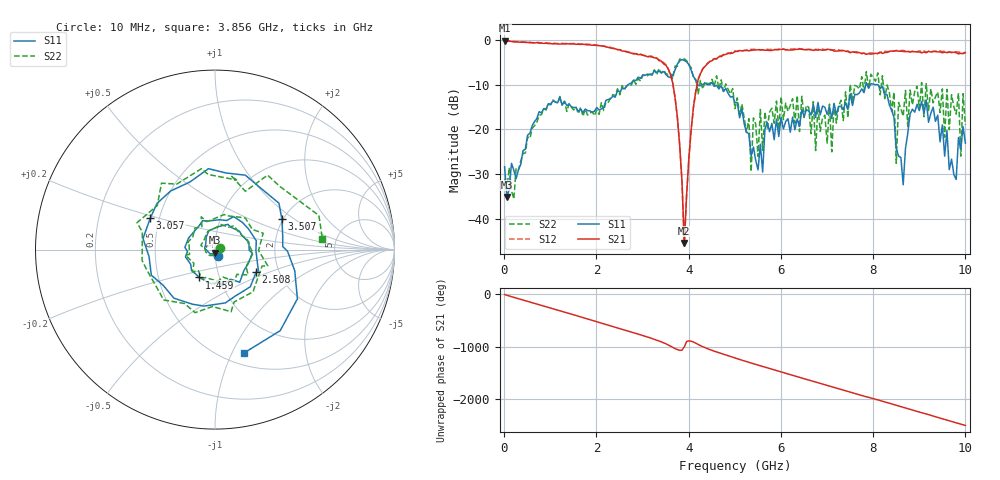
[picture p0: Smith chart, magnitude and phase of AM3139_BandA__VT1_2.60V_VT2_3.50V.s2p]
! Date/Time: Tue, Nov 13, 2018 4:57 PM
! Network Analyzer: Agilent Technologies E8364B Rev: A.07.50.67
! Sweep from 0.010 to 10.000 GHz, 201 Points, Sweep Type: LIN
! Power Supply: 2.601 V, 0.000 A
# Hz S DB R 50
!freq MagS11 AngS11 MagS21 AngS21 MagS12 AngS12 MagS22 AngS22
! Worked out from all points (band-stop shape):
!   201 points, 10 MHz to 10 GHz, reference 50 ohm
!   highest |S21| = -0.23 dB at 10 MHz (marker M1); lowest = -45.3 dB at 3.906 GHz (marker M2)
!   |S21| within 3 dB of the highest: start of sweep to 2.874 GHz; 4.816 GHz to 7.843 GHz (3.027 GHz wide, 47.8 % of centre)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
!   lowest |S11| = -35.1 dB at 59.95 MHz (marker M3), VSWR 1.04, Z = 49.8 - j1.75 ohm
!   |S11| at or under -10 dB: start of sweep to 2.696 GHz; 4.531 GHz to 7.843 GHz (3.312 GHz wide, 53.5 % of centre); 8.036 GHz to end of sweep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
!   |S22| runs from -35.5 to -4.3 dB; largest |S21 - S12| = 0.034
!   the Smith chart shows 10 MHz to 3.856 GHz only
!   S11 on the Smith chart (normalised r, x): 10 MHz: 1.03, -0.07; 1.459 GHz: 0.80, -0.26; 2.508 GHz: 1.53, -0.41; 3.057 GHz: 0.45, +0.19; 3.507 GHz: 1.97, +0.80; 3.856 GHz: 0.62, -1.11
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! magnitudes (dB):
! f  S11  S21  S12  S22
! 10 MHz  -28.3  -0.2  -0.2  -31.0
! 59.95 MHz  -35.1  -0.3  -0.2  -33.3
! 1.459 GHz  -15.0  -0.9  -0.9  -15.1
! 1.708 GHz  -16.3  -1.0  -1.0  -17.1
! 2.508 GHz  -11.7  -2.3  -2.2  -12.3
! 3.057 GHz  -7.9  -3.6  -3.6  -8.1
! 3.357 GHz  -7.0  -4.7  -4.5  -6.5
! 3.507 GHz  -7.8  -5.7  -5.5  -7.5
! 3.856 GHz  -4.5  -31.7  -31.7  -4.4
! 3.906 GHz  -4.6  -45.3  -46.0  -4.3
! 4.206 GHz  -10.2  -8.9  -8.8  -12.1
! 5.005 GHz  -14.0  -2.7  -2.5  -15.4
! 5.604 GHz  -29.5  -2.3  -2.3  -24.7
! 6.703 GHz  -14.5  -2.4  -2.3  -13.8
! 7.103 GHz  -17.6  -2.3  -2.3  -25.0
! 7.502 GHz  -12.1  -2.9  -2.8  -10.0
! 8.352 GHz  -14.6  -2.6  -2.7  -11.8
! 8.452 GHz  -17.3  -2.6  -2.6  -11.7
! 8.501 GHz  -24.3  -2.5  -2.4  -27.6
! 8.651 GHz  -32.3  -2.6  -2.4  -17.0
! 8.951 GHz  -14.4  -2.7  -2.7  -10.4
! 10 GHz  -23.1  -2.9  -2.8  -19.0
